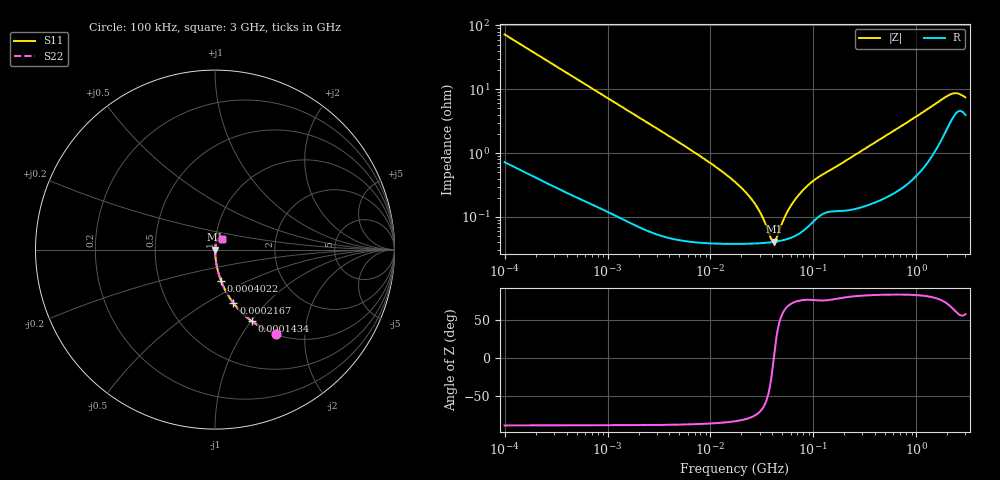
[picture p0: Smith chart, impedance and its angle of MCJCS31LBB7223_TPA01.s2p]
! MCJCS31LBB7223_TPA01  S-PARAMETER MODEL  ( Standard Model )
! Model Generated by TAIYO YUDEN Corporation (http://www.ty-top.com)
! Version 1.0
! TAIYO YUDEN Control No. 220601
! Copyright(c) 2015 TAIYO YUDEN CO.,LTD. All Rights Reserved.
! Product Description (link to TY-COMPAS)
! https://ds.yuden.co.jp/TYCOMPAS/or/detail?pn=MCJCS31LBB7223KTPA01&u=M
! Products Name : Multilayer Ceramic Capacitors
! Characteristics :
!  Capacitance : 0.022 [uF] , Rated Voltage : 630 [V] , TCC : X7R
!  Case Size : 3.2 x 1.6 / 0.126 x 0.063 [mm/inch] , Thickness : 1.6 / 0.063 [mm/inch]
!  (Conditions: Temperature = 25 [degC] , DC Bias Voltage = 0 [V])
! External Node Assignments :
!  1  o---| |---o  2
! GND o---------o GND
! Frequency Range : 100kHz  -  3GHz  [ 401 STEP ]
# MHZ S RI R 50
! Freq[MHz].  S11 Real  S11 Imag  S21 Real  S21 Imag  S12 Real  S12 Imag  S22 Real  S22 Imag
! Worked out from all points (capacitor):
!   401 points, 100 kHz to 3 GHz, reference 50 ohm
!   read as one part in series: C = 22.1 nF near 105.3 kHz
!   lowest |Z| = 41 mohm at 41.6 MHz (marker M1)
!   series resonance near 41.24 MHz, so ESL is about 670 pH
!   S11 on the Smith chart (normalised r, x): 100 kHz: 1.01, -1.44; 143.4 kHz: 1.01, -1.01; 216.7 kHz: 1.01, -0.67; 402.2 kHz: 1.00, -0.36; 3 GHz: 1.08, +0.13
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0.1  0.3425 -0.4695  0.6575 0.4695  0.6575 0.4695  0.3425 -0.4695
0.14345  0.2042 -0.3978  0.7958 0.3978  0.7958 0.3978  0.2042 -0.3978
0.216663  0.103 -0.2982  0.897 0.2982  0.897 0.2982  0.103 -0.2982
0.402172  0.0337 -0.1741  0.9663 0.1741  0.9663 0.1741  0.0337 -0.1741
0.562235  0.0183 -0.1269  0.9817 0.1269  0.9817 0.1269  0.0183 -0.1269
3.161081  0.00106 -0.0232  0.9989 0.0232  0.9989 0.0232  0.00106 -0.0232
9.574722  0.000441 -0.0073  0.9996 0.0073  0.9996 0.0073  0.000441 -0.0073
17.7727  0.00039 -0.00339  0.9996 0.00339  0.9996 0.00339  0.00039 -0.00339
22.99754  0.000386 -0.00222  0.9996 0.00222  0.9996 0.00222  0.000386 -0.00222
27.54426  0.000387 -0.00149  0.9996 0.00149  0.9996 0.00149  0.000387 -0.00149
32.15051  0.000392 -0.000906  0.9996 0.000906  0.9996 0.000906  0.000392 -0.000906
38.50681  0.000402 -0.000248  0.9996 0.000248  0.9996 0.000248  0.000402 -0.000248
41.60216  0.000408 3.16e-05  0.9996 -3.16e-05  0.9996 -3.16e-05  0.000408 3.16e-05
43.80277  0.000413 0.000218  0.9996 -0.000218  0.9996 -0.000218  0.000413 0.000218
52.46276  0.00044 0.000881  0.9996 -0.000881  0.9996 -0.000881  0.00044 0.000881
61.23616  0.000479 0.00148  0.9995 -0.00148  0.9995 -0.00148  0.000479 0.00148
75.25761  0.000574 0.00233  0.9994 -0.00233  0.9994 -0.00233  0.000574 0.00233
97.38194  0.000825 0.00348  0.9992 -0.00348  0.9992 -0.00348  0.000825 0.00348
547.5153  0.00254 0.02  0.9975 -0.02  0.9975 -0.02  0.00254 0.02
2038.117  0.0305 0.0712  0.9695 -0.0712  0.9695 -0.0712  0.0305 0.0712
2441.062  0.0456 0.0693  0.9544 -0.0693  0.9544 -0.0693  0.0456 0.0693
3000  0.0416 0.0584  0.9584 -0.0584  0.9584 -0.0584  0.0416 0.0584
